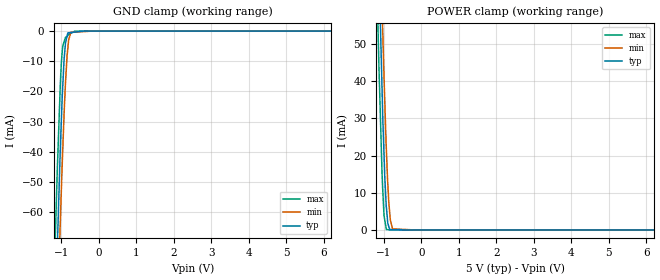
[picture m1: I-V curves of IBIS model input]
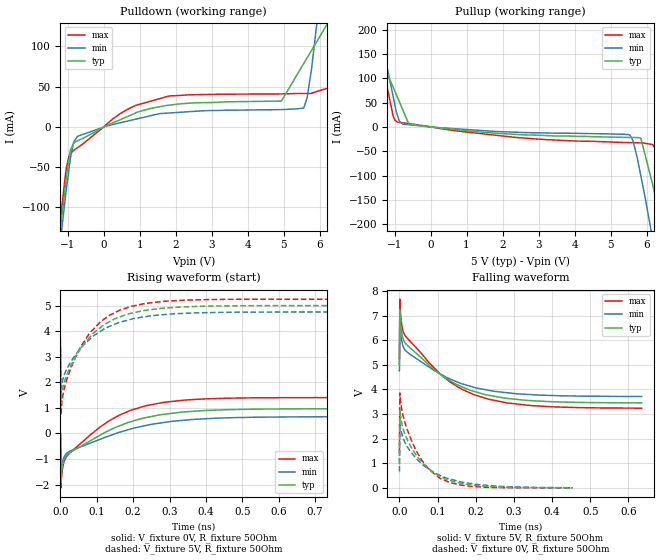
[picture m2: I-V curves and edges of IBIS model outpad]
|Texas Instruments Incorporated
|16-Bit, Dual Voltage Output DAC with Serial Interface
| Marketing part#   Digital Voltage Range   Package-type   #pins
| DAC7632VFBT   4.75V - 5.25V   LQFP   32
| DAC7632VFBTG4   4.75V - 5.25V   LQFP   32
| DAC7632VFR   4.75V - 5.25V   LQFP   32
| DAC7632VFRG4   4.75V - 5.25V   LQFP   32
| DAC7632VFT   4.75V - 5.25V   LQFP   32
| DAC7632VFTG4   4.75V - 5.25V   LQFP   32
[IBIS Ver]   3.2
[File name]   dac7632.ibs
|SIMDE Ver   V2.2 - 201009 - Build - 424
[File Rev]   1.0
[Date]   11/ 9/ 2011
[Source]
| Texas Instruments Incorporated.
| Analog-eLab Design Center, HPA
| 12500 TI Blvd
| Dallas, TX -75243
| e-mail: elab_scm_ibis@list.ti.com
[Notes]   Revision History:
| Rev 1.0: 11/9/2011
| - Initial version of the model
| - Model generated from simulations in SPECTRE
| - Model matched to SPICE simulation
| - C_comp although listed in numerical order of value are
|   obtained from varying PVT conditions. For PVT conditions for
|   each specific value refer the buffer description under
|   respective [Model]. IBIS model user is responsible for using
|   appropriate C_comp to simulate for Signal Integrity.
| - Model names with a trailing _5 contains the model for
|   5V [4.75V and 5.25V].
[Disclaimer]
| This model is designed as an aid for customers of Texas Instruments.
| TI and its licensors and suppliers make no warranties, either expressed
| or implied, with respect to this  model, including the warranties of
| merchantability or fitness for a particular purpose. The model is
| provided solely on an "as is" basis. The entire risk as to its quality
| and performance is with the customer.
[Copyright]
 (C) Copyright 2011 Texas Instruments Incorporated.All rights reserved.
|   DAC7632VF
[Component]   DAC7632VF
[Manufacturer]   TI
[Package]   |32 LQFP - VF package
|   typ   min   max
R_pkg   0.08106   0.07839   0.08651
L_pkg   2.54808nH   2.37787nH   2.80852nH
C_pkg   0.37291pF   0.34231pF   0.39520pF
[Pin]  signal_name   model_name   R_pin   L_pin   C_pin
1   VCC   POWER   0.08007   2.68878nH  0.37729pF
2   AGND   GND   0.07771   2.50957nH  0.39264pF
3   AGND   GND   0.08255   2.47328nH  0.38152pF
4   NC   NC   0.00350   1.19747nH  0.26734pF
5   DGND   GND   0.08309   2.47291nH  0.34833pF
6   DGND   GND   0.07981   2.42035nH  0.38008pF
7   VDD   POWER   0.07921   2.54038nH  0.38914pF
8   SDO   outpad   0.08135   2.71415nH  0.37691pF
9   NC   NC   0.00424   1.48778nH  0.30265pF
10   NC   NC   0.00398   1.34757nH  0.31551pF
11   NC   NC   0.00354   1.20728nH  0.30102pF
12   NC   NC   0.00350   1.19747nH  0.26734pF
13   NC   NC   0.00350   1.19815nH  0.26717pF
14   NC   NC   0.00354   1.20789nH  0.30078pF
15   NC   NC   0.00398   1.34770nH  0.31544pF
16   NC   NC   0.00421   1.48381nH  0.30322pF
17   CLK   input   0.08159   2.72208nH  0.37661pF
18   SDI   input   0.07938   2.54327nH  0.38973pF
19   _CS   input   0.07965   2.41598nH  0.37596pF
20   RSTSEL   input   0.08129   2.43837nH  0.34334pF
21   RST   input   0.08138   2.44045nH  0.34325pF
22   LDAC   input   0.07993   2.42119nH  0.37581pF
23   _LOAD   input   0.07950   2.54350nH  0.38973pF
24   VSS   TERM   0.08156   2.71411nH  0.37893pF
25   VOUTB   TERM   0.08291   2.74178nH  0.37929pF
26   VOUTBSense   TERM   0.08173   2.58357nH  0.39222pF
27   VREFHSense   TERM   0.07865   2.39208nH  0.37623pF
28   VREFH   TERM   0.07839   2.37787nH  0.34231pF
29   VREFL   TERM   0.07904   2.39106nH  0.34286pF
30   VREFLSense   TERM   0.08046   2.42769nH  0.37796pF
31   VREFASense   TERM   0.08471   2.64171nH  0.39520pF
32   VOUTA   TERM   0.08651   2.80852nH  0.38315pF
[Model] TERM
Model_type Terminator
C_comp   1.0e-20F  1.0e-20F  1.0e-20F
|   typ   min   max
[Voltage Range]   5V   4.75V   5.25V
[POWER Clamp Reference]   5V   4.75V   5.25V
[GND Clamp Reference]   0V   0V   0V
|Ambient Temperature   25   85   -40
|Junction Temperature
[Temperature Range]   25   85   -40
| Models and submodels in the file (3): input (Input), outpad (Output), TERM (Terminator)
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|   input Model
[Model]   input
Model_type   Input
Vinl = 1.5
Vinh = 3.5
|   typ   min   max
|C_comp from frequency sweep method (F= 20 MHz)
C_comp   2.146e-12   2.146e-12   2.149e-12
|C_comp (ON state)   2.146e-12   2.149e-12   2.146e-12
|C_comp (OFF state)   2.146e-12   2.149e-12   2.146e-12
|C_comp from LC Tank method (L = 1nH)
|Resonant Frequency(Hz)   3.050e+09   2.990e+09  3.110e+09
|C_comp   2.726e-12   2.836e-12  2.622e-12
| Where nom  PVT is Nominal Process, 5V, 25C
|   Fast PVT is Strong Process,  5.25V, -40C
|   Slow PVT is Weak Process,   4.75V, 85C
[Model Spec]
|Subparameter   typ   min   max
Vinh   3.5   3.325   3.675
Vinl   1.5   1.425   1.575
[Voltage Range]   5   4.75   5.25
|Ambient Temperature   25   85   -40
|Junction Temperature
[Temperature Range]   25   85   -40
[Power Clamp Reference]   5   4.75   5.25
[GND Clamp Reference]   0   0   0
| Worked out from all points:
|   GND clamp passes 1 mA (typ) near -0.83 V on its own axis
|   POWER clamp passes 1 mA (typ) near -0.87 V on its own axis
[GND Clamp]
|   Voltage   I(typ)   I(min)   I(max)
-5V       -1.943A    -1.95A     -1.934A
-1.246V   -129.5mA   -154.5mA   -105.1mA
-1.11V    -73.07mA   -96.12mA   -46.89mA
-1.062V   -53.44mA   -76.78mA   -30.12mA
-1.031V   -40.53mA   -64.82mA   -19.1mA
-994.2mV  -27.96mA   -50.75mA   -9.598mA
-925mV    -9.074mA   -27.29mA   -3.512mA
-889.2mV  -4.038mA   -17.26mA   -2.076mA
-825mV    -591.9uA   -5.505mA   -1.427mA
-748.8mV  -488.2uA   -420.5uA   -775.3uA
-174mV    0A         0A         0A
10V       0A         0A         0A
[POWER Clamp]
|   Voltage   I(typ)   I(min)   I(max)
-5V       1.891A     1.904A     1.884A
-1.246V   116.9mA    141.5mA    91.87mA
-1.131V   71.04mA    93.83mA    44.09mA
-1.072V   47.62mA    69.46mA    23.65mA
-1.03V    31.05mA    53.94mA    10.96mA
-994.2mV  20.16mA    41.11mA    3.819mA
-975mV    14.48mA    34.81mA    2.693mA
-931.3mV  5.978mA    21.37mA    133.4uA
-862.8mV  738.8uA    6.6mA      54.29uA
-824.7mV  114.9uA    2.553mA    10.4uA
-767.8mV  99.81uA    303.5uA    0A
10V       0A         0A         0A
|   outpad Model
[Model]   outpad
Model_type   Output
Polarity   Inverting
Vmeas = 2.5
Vref = 2.5
Cref = 2pF
Rref = 50
|   typ   min   max
|C_comp from frequency sweep method (F=16.67 MHz)
C_comp   2.080e-12   2.053e-12   2.083e-12
|C_comp (ON state)   2.080e-12   2.053e-12   2.083e-12
|C_comp (OFF state)   2.005e-12   1.994e-12   1.996e-12
|C_comp from LC Tank method (L = 1nH)
|resonant_f(ON)   3.100e+09   3.040e+09   3.180e+09
|C_comp(ON)   2.638e-12   2.744e-12   2.507e-12
|resonant_f(OFF)   3.040e+09   2.980e+09   3.100e+09
|C_comp(OFF)   2.744e-12   2.855e-12   2.638e-12
| Where nom  PVT is Nominal Process, 5V, 25C
|   Fast PVT is Strong Process,  5.25V, -40C
|   Slow PVT is Weak Process,   4.75V, 85C
[Voltage Range]   5   4.75   5.25
|Ambient Temperature   25   85   -40
|Junction Temperature
[Temperature Range]   25   85   -40
[Pullup Reference]   5   4.75   5.25
[Pulldown Reference]   0   0   0
[Power Clamp Reference]   5   4.75   5.25
[GND Clamp Reference]   0   0   0
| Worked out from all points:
|   slope of the pulldown table from 0 to 0.75 V, typ, clamps not added: 51.6 ohm
|   slope of the pullup table from 0 to 0.75 V, typ, clamps not added: 134 ohm
|   falling waveform, V_fixture 5V, R_fixture 50Ohm: 20-80 % time 133ps typ, 132ps min, 133ps max; typ from 5 V to 3.45 V
|   rising waveform, V_fixture 0V, R_fixture 50Ohm: 20-80 % time 154ps typ, 165ps min, 138ps max; typ from 0 V to 0.968 V
|   rising waveform, V_fixture 5V, R_fixture 50Ohm: 20-80 % time 112ps typ, 121ps min, 102ps max; typ from 3.45 V to 5 V
|   falling waveform, V_fixture 0V, R_fixture 50Ohm: 20-80 % time 82.2ps typ, 100ps min, 64.1ps max; typ from 0.968 V to 0.001 V
[Pulldown]
|   Voltage   I(typ)   I(min)   I(max)
-5V       -1.831A    -1.827A    -1.825A
-1.243V   -143.7mA   -158.6mA   -131.3mA
-952.3mV  -37.27mA   -48.98mA   -34.38mA
-720.2mV  -17.01mA   -11.57mA   -25.57mA
664.7mV   12.9mA     7.288mA    21.86mA
1.82V     27.1mA     17.33mA    38.5mA
4.935V    32.11mA    21.5mA     41.03mA
5.554V    78.62mA    23.48mA    41.56mA
5.778V    95.42mA    73.49mA    42.08mA
6.2V      127.1mA    237mA      47.9mA
6.561V    273.7mA    390.1mA    157.6mA
10V       1.788A     1.889A     1.694A
[Pullup]
|   Voltage   I(typ)   I(min)   I(max)
-5V       1.748A     1.758A     1.739A
-2.296V   563.5mA    581mA      547.1mA
-1.25V    118.4mA    139mA      98.31mA
-994.2mV  73.95mA    46.71mA    14.17mA
-767.8mV  34.56mA    5.413mA    8.297mA
0V        0A         0A         0A
5.526V    -21.6mA    -15.9mA    -32.24mA
5.84V     -22.97mA   -100.1mA   -32.79mA
6.172V    -118.9mA   -231.7mA   -36.16mA
6.508V    -255.1mA   -375.7mA   -139.2mA
6.76V     -362mA     -485mA     -248.2mA
10V       -1.811A    -1.919A    -1.702A
[Ramp]
R_load = 50
|   typ   min   max
dV/dt_r   0.580857/1.53933e-10   0.395191/1.64703e-10   0.842654/1.37799e-10
dV/dt_f   0.930566/1.33861e-10   0.624794/1.54954e-10   1.21095/1.34024e-10
[Falling Waveform]
V_fixture = 5V
V_fixture_min = 4.75V
V_fixture_max = 5.25V
R_fixture = 50Ohm
|   Time   V(typ)   V(min)   V(max)
0s        5V         4.75V      5.25V
1ps       7.234V     6.824V     7.667V
3.225ps   6.684V     6.331V     7.043V
6.074ps   6.292V     5.972V     6.612V
16.23ps   5.865V     5.574V     6.154V
107.6ps   4.611V     4.624V     4.612V
162.5ps   4.114V     4.235V     4.015V
234.8ps   3.759V     3.962V     3.597V
344ps     3.544V     3.789V     3.345V
634.7ps   3.453V     3.713V     3.237V
[Rising Waveform]
V_fixture = 0V
V_fixture_min = 0V
V_fixture_max = 0V
R_fixture = 50Ohm
|   Time   V(typ)   V(min)   V(max)
0s        110.1pV    133.9pV    85.15pV
1ps       -1.926V    -1.748V    -2.125V
3.225ps   -1.522V    -1.373V    -1.673V
6.074ps   -1.231V    -1.106V    -1.342V
16.23ps   -870.5mV   -789.7mV   -912.7mV
107.6ps   -77.7mV    -235.7mV   239.3mV
194.8ps   465.4mV    182.2mV    913.8mV
344ps     846.2mV    522.6mV    1.309V
726.3ps   964.6mV    654.7mV    1.401V
3ns       968.1mV    658.7mV    1.404V
[Rising Waveform]
V_fixture = 5V
V_fixture_min = 4.75V
V_fixture_max = 5.25V
R_fixture = 50Ohm
|   Time   V(typ)   V(min)   V(max)
0s        3.449V     3.709V     3.232V
1ps       1.147V     1.582V     722.8mV
7.916ps   1.867V     2.185V     1.582V
20.4ps    2.386V     2.598V     2.231V
42.87ps   3.028V     3.101V     3.027V
79.18ps   3.736V     3.664V     3.898V
107.6ps   4.113V     3.968V     4.335V
162.5ps   4.55V      4.344V     4.815V
284.3ps   4.898V     4.645V     5.164V
3ns       5V         4.75V      5.25V
[Falling Waveform]
V_fixture = 0V
V_fixture_min = 0V
V_fixture_max = 0V
R_fixture = 50Ohm
|   Time   V(typ)   V(min)   V(max)
0s        968.1mV    658.7mV    1.404V
1ps       3.163V     2.632V     3.857V
6.074ps   2.628V     2.202V     3.199V
12.91ps   2.249V     1.898V     2.734V
42.87ps   1.356V     1.217V     1.54V
79.18ps   748.2mV    742.3mV    715.9mV
107.6ps   464mV      504.7mV    379.2mV
162.5ps   185.8mV    236.3mV    108.6mV
225.7ps   62.38mV    108mV      27.2mV
454.7ps   1.225mV    6.314mV    1.171mV
